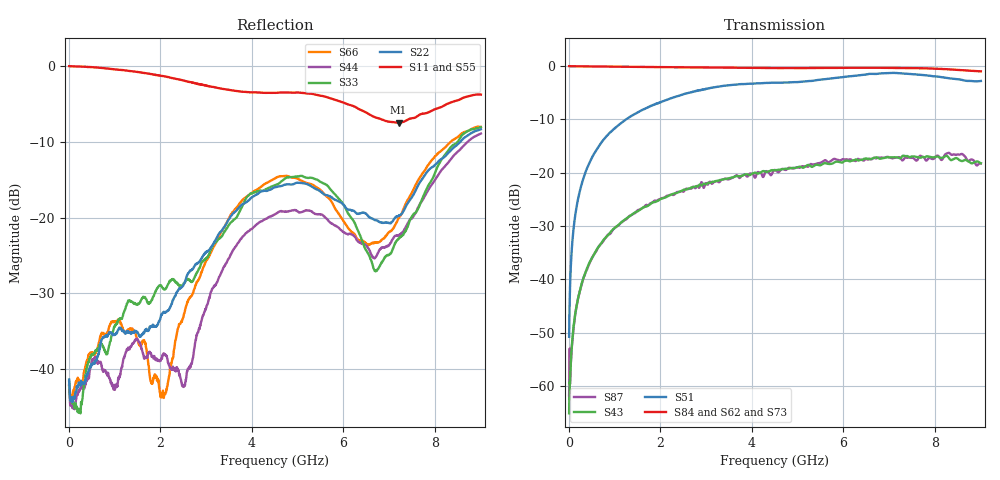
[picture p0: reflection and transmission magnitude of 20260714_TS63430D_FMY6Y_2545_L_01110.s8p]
# GHz S DB R 50
! CMT, SN0916, 25263762, 26.7.0
! Date: 15.07.2026 14:59:25
! Data: Format
! Freq S1.1:dB/Ang S1.2:dB/Ang S1.3:dB/Ang S1.4:dB/Ang S1.5:dB/Ang S1.6:dB/Ang S1.7:dB/Ang S1.8:dB/Ang
!  S2.1:dB/Ang S2.2:dB/Ang S2.3:dB/Ang S2.4:dB/Ang S2.5:dB/Ang S2.6:dB/Ang S2.7:dB/Ang S2.8:dB/Ang
!  S3.1:dB/Ang S3.2:dB/Ang S3.3:dB/Ang S3.4:dB/Ang S3.5:dB/Ang S3.6:dB/Ang S3.7:dB/Ang S3.8:dB/Ang
!  S4.1:dB/Ang S4.2:dB/Ang S4.3:dB/Ang S4.4:dB/Ang S4.5:dB/Ang S4.6:dB/Ang S4.7:dB/Ang S4.8:dB/Ang
!  S5.1:dB/Ang S5.2:dB/Ang S5.3:dB/Ang S5.4:dB/Ang S5.5:dB/Ang S5.6:dB/Ang S5.7:dB/Ang S5.8:dB/Ang
!  S6.1:dB/Ang S6.2:dB/Ang S6.3:dB/Ang S6.4:dB/Ang S6.5:dB/Ang S6.6:dB/Ang S6.7:dB/Ang S6.8:dB/Ang
!  S7.1:dB/Ang S7.2:dB/Ang S7.3:dB/Ang S7.4:dB/Ang S7.5:dB/Ang S7.6:dB/Ang S7.7:dB/Ang S7.8:dB/Ang
!  S8.1:dB/Ang S8.2:dB/Ang S8.3:dB/Ang S8.4:dB/Ang S8.5:dB/Ang S8.6:dB/Ang S8.7:dB/Ang S8.8:dB/Ang
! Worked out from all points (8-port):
!   2001 points, 10 MHz to 9 GHz, reference 50 ohm
!   strongest paths, dB at 10 MHz, 2.257 GHz, 4.505 GHz, 6.753 GHz, 9 GHz:
!     S84: -0.1, -0.3, -0.4, -0.4, -1.0
!     S62: -0.1, -0.3, -0.5, -0.4, -1.2
!     S73: -0.1, -0.3, -0.6, -0.4, -1.2
!     S51: -50.8, -6.0, -3.2, -1.5, -2.9
!     S43: -65.1, -24.1, -19.6, -17.3, -18.3
!     S87: -61.7, -24.2, -19.5, -17.2, -18.3
!   lowest |S11| = -7.5 dB at 7.202 GHz (marker M1), VSWR 2.47, Z = 21.1 - j9.28 ohm
!   |S11| at or under -10 dB: nowhere
